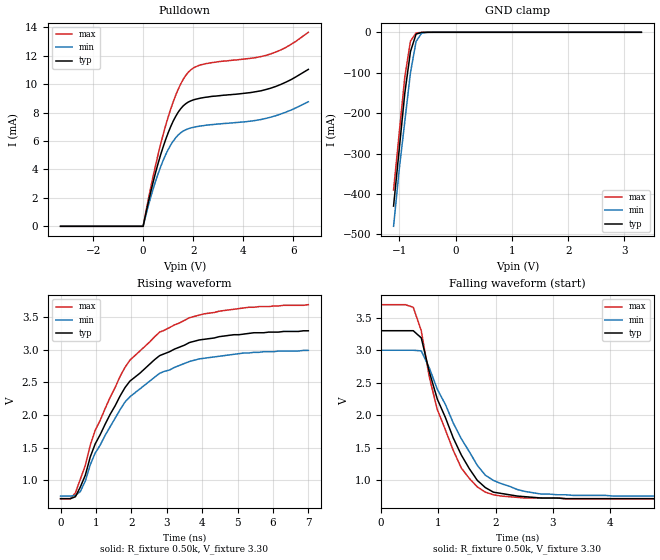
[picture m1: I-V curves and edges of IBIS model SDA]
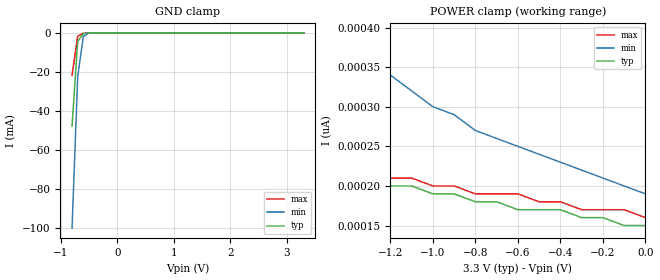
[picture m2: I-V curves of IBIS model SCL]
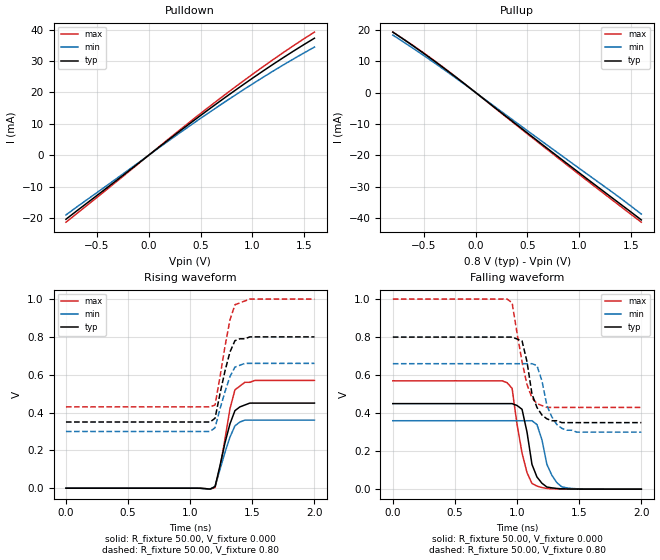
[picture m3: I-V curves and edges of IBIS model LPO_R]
| Integrated Devices Technolgy, Inc
[Ibis Ver]   3.2
[File Name]   9eprs488.ibs
[File Rev]   1.0
[Date]   08/18/2010
[Source]   Integrated Devices Technolgy, Inc.
[Notes]   Rev 0.0 created by ss
[Disclaimer] Integrated Device Technology, Inc. ("IDT") hereby grants the
   user of this IBIS model a non-exclusive, nontransferable
   license to use this IBIS model under the following terms. The
   user is granted this license only to use the IBIS model and is
   not granted rights to sell, copy (except as needed to run the
   IBIS model), rent, lease or sub-license the IBIS model in
   whole or in part, or in modified form to anyone. The User may
   modify the IBIS model to suit its specific applications, but
   rights to derivative works and such modifications shall belong
   to IDT. This IBIS model is provided on an AS IS" basis and IDT
   makes absolutely no warranty with respect to the information
   contained herein. IDT DISCLAIMS AND CUSTOMER WAIVES ALL
   WARRANTIES, EXPRESS AND IMPLIED, INCLUDING WARRANTIES OF
   MERCHANTABILITY AND FITNESS FOR A PARTICULAR PURPOSE. THE
   ENTIRE RISK AS TO QUALITY AND PERFORMANCE IS WITH THE USER
   ACCORDINGLY, IN NO EVENT SHALL IDT BE LIABLE FOR ANY DIRECT OR
   INDIRECT DAMAGES, WHETHER IN CONTRACT OR TORT, INCLUDING ANY
   LOST PROFITS OR OTHER INCIDENTAL, CONSEQUENTIAL, EXEMPLARY, OR
   PUNITIVE DAMAGES ARISING OUT OF THE USE OR APPLICATION OF THE
   IBIS model. Further, IDT reserves the right to make changes
   without notice to any product herein to improve reliability,
   function, or design. IDT does not convey any license under
   patent rights or any other intellectual property rights,
   including those of third parties. IDT is not obligated to
   provide maintenance or support for the licensed IBIS model.
[Copyright]   Copyright 2006, Integrated Devices Technolgy, Inc. all rights
   reserved
|   COMPONENT: ICS9LPRS4888
[Component]   IDT9LPRS488
[Manufacturer]   Integrated Device Technology, Inc.
[Package]
| variable   typ   min   max
R_pkg   81.1m   62.2m   100.0m
L_pkg   6.7nH   4.9nH   8.5nH
C_pkg   0.53pF   0.21pF   0.85pF
[Pin]  signal_name   model_name   R_pin   L_pin   C_pin
1   SMBCLK   SCL
2   SMBDAT   SDA
3   VDD   POWER
4   SRC7C_LPRS/27MHz_NS   LPO_R
5   SRC7T_LPRS/27MHz_SS   LPO_R
6   GND   GND
7   SRC5C_LPRS   LPO_R
8   SRC5T_LPRS   LPO_R
9   SRC4C_LPRS   LPO_R
10   SRC4T_LPRS   LPO_R
11   GNDSRC   GND
12   VDDSRC_IO   POWER
13   SRC3C_LPRS   LPO_R
14   SRC3T_LPRS   LPO_R
15   SRC2C_LPRS   LPO_R
16   SRC2T_LPRS   LPO_R
17   VDDSRC   POWER
18   VDDSRC_IO   POWER
19   GNDSRC   GND
20   SRC1C_LPRS   LPO_R
21   SRC1T_LPRS   LPO_R
22   SRC0C_LPRS   LPO_R
23   SRC0T_LPRS   LPO_R
24   **CLKREQ0#   IN_PD
25   ATIG2C_LPRS   LPO_R
26   ATIG2T_LPRS   LPO_R
27   GNDATIG   GND
28   VDDATIG_IO   POWER
29   VDDATIG   POWER
30   ATIG1C_LPRS   LPO_R
31   ATIG1T_LPRS   LPO_R
32   ATIG0C_LPRS   LPO_R
33   ATIG0T_LPRS   LPO_R
34   SB_SRC1C_LPRS   LPO_R
35   SB_SRC1T_LPRS   LPO_R
36   GNDSB_SRC   GND
37   VDDSB_SRC_IO   POWER
38   VDDSB_SRC   POWER
39   SB_SRC0C_LPRS   LPO_R
40   SB_SRC0T_LPRS   LPO_R
41   SB_SRC_SLOW#*   IN_PU
42   CLKREQ4#**   IN_PD
43   CLKREQ3#**   IN_PD
44   VDDSATA   POWER
45   SRC6C/SATAC_LPRS   LPO_R
46   SRC6T/SATAT_LPRS   LPO_R
47   GNDSATA   GND
48   GNDA   GND
49   VDDA   POWER
50   CLKREQ2#**   IN_PD
51   CLKREQ1#**   IN_PD
52   GNDCPU   GND
53   VDDCPU_IO   POWER
54   VDDCPU   POWER
55   CPUKG0C_LPR   LPO_R
56   CPUKG0T_LPRS   LPO_R
57   PD#   IN
58   GNDHTT   GND
59   HTT0C_LPRS/66M   LPO_R
60   HTT0T_LPRS/66M   LPO_R
61   VDDHTT   POWER
62   VDDREF   POWER
63   REF2/SEL_27   SE_2X_SR
64   REF1/SEL_SATA   SE_2X_SR
65   REF0/SEL_HTT66   SE_2X_SR
66   GNDREF   GND
67   X1   XT1
68   X2   XTL_OUT
69   VDD48   POWER
70   48MHz_1   SE_2X_SR
71   48MHz_0   SE_2X_SR
72   GND48   GND
[Diff Pin]   inv_pin   vdiff   tdelay_typ   tdelay_min   tdelay_max
5   4   NA   NA
8   7   NA   NA
10   9   NA   NA
14   13   NA   NA
16   15   NA   NA
21   20   NA   NA
23   22   NA   NA
26   25   NA   NA
31   30   NA   NA
33   32   NA   NA
35   34   NA   NA
40   39   NA   NA
46   45   NA   NA
56   55   NA   NA
60   59   NA   NA
| Models and submodels in the file (9): SDA (I/O_open_drain), SCL (Input), LPO_R (Output), XT1 (Input), IN (Input), SE_2X_SR (Output), IN_PD (Input), IN_PU (Input), XTL_OUT (Output)
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|   Model SDA
[Model]   SDA
Model_type   I/O_open_drain
Polarity   Inverting
Enable   Active-High
Vinl =   0.80V
Vinh =   2.00V
Vmeas =   1.50V
Cref =   5.00pF
Rref =  0.000
Vref =   1.50V
C_comp   3.40pF   2.85pF   3.95pF
[Temperature Range]   27.00   70.00   0.000
[Voltage Range]   3.30V   3.00V   3.70V
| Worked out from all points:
|   slope of the pulldown table from 0 to 0.495 V, typ, clamps not added: 131 ohm
|   GND clamp passes 1 mA (typ) near -0.62 V on its own axis
|   rising waveform, R_fixture 0.50k, V_fixture 3.30: 20-80 % time 1.74ns typ, 1.76ns min, 1.73ns max; typ from 0.72 V to 3.29 V
|   falling waveform, R_fixture 0.50k, V_fixture 3.30: 20-80 % time 693ps typ, 785ps min, 596ps max; typ from 3.3 V to 0.72 V
[Pulldown]
| voltage   I(typ)   I(min)   I(max)
-3.3V     0A         0A         0A
0V        0A         0A         0A
500mV     3.8mA      3.19mA     4.32mA
900mV     6.11mA     5.04mA     7.1mA
1.2V      7.4mA      5.99mA     8.75mA
1.4V      8.03mA     6.42mA     9.64mA
1.8V      8.74mA     6.86mA     10.83mA
2.1V      8.94mA     7mA        11.22mA
2.5V      9.08mA     7.11mA     11.44mA
5.1V      9.72mA     7.68mA     12.13mA
5.7V      10.14mA    8.03mA     12.58mA
6.6V      11.04mA    8.76mA     13.65mA
[GND_clamp]
| voltage   I(typ)   I(min)   I(max)
  |-3.30   -3.78A   -3.64A   -3.87A
  |-3.20   -3.62A   -3.50A   -3.71A
  |-3.10   -3.47A   -3.35A   -3.55A
  |-3.00   -3.31A   -3.21A   -3.39A
  |-2.90   -3.16A   -3.06A   -3.23A
  |-2.80   -3.01A   -2.91A   -3.07A
  |-2.70   -2.85A   -2.77A   -2.91A
  |-2.60   -2.70A   -2.62A   -2.75A
  |-2.50   -2.54A   -2.48A   -2.59A
  |-2.40   -2.39A   -2.33A   -2.43A
  |-2.30   -2.24A   -2.19A   -2.27A
  |-2.20   -2.08A   -2.04A   -2.11A
  |-2.10   -1.93A   -1.90A   -1.95A
  |-2.00   -1.78A   -1.75A   -1.79A
  |-1.90   -1.62A   -1.61A   -1.63A
  |-1.80   -1.47A   -1.46A   -1.47A
  |-1.70   -1.32A   -1.32A   -1.32A
  |-1.60   -1.17A   -1.18A   -1.16A
  |-1.50   -1.02A   -1.03A   -1.00A
  |-1.40   -0.87A   -0.89A   -0.85A
  |-1.30   -0.72A   -0.75A   -0.69A
  |-1.20   -0.57A   -0.61A   -0.54A
-1.1V     -430mA     -480mA     -390mA
-1V       -290mA     -340mA     -250mA
-900mV    -150mA     -220mA     -110mA
-800mV    -47.73mA   -100mA     -21.74mA
-700mV    -4.4mA     -22.46mA   -1.7mA
-600mV    -390uA     -1.82mA    -190uA
-400mV    -1.59uA    -9.25uA    -420nA
3.3V      150pA      220pA      150pA
[Ramp]
| variable   typ   min   max
dV/dt_r   0.27/0.19n   0.21/0.19n   0.35/0.18n
dV/dt_f   0.27/0.21n   0.21/0.22n   0.35/0.20n
[Rising Waveform]
R_fixture = 0.50k
V_fixture = 3.30
V_fixture_min = 3.00
V_fixture_max = 3.70
| time   V(typ)   V(min)   V(max)
0s        720mV      760mV      720mV
280ps     720mV      760mV      720mV
420ps     750mV      770mV      810mV
560ps     900mV      830mV      1.02V
700ps     1.08V      990mV      1.23V
980ps     1.56V      1.42V      1.77V
1.82ns    2.42V      2.2V       2.73V
2.8ns     2.91V      2.64V      3.27V
4.06ns    3.16V      2.87V      3.55V
7ns       3.29V      2.99V      3.69V
[Falling Waveform]
R_fixture = 0.50k
V_fixture = 3.30
V_fixture_min = 3.00
V_fixture_max = 3.70
| time   V(typ)   V(min)   V(max)
0s        3.3V       3V         3.7V
560ps     3.3V       3V         3.66V
700ps     3.19V      2.99V      3.3V
840ps     2.67V      2.73V      2.59V
980ps     2.25V      2.4V       2.09V
1.4ns     1.39V      1.64V      1.19V
1.68ns    1V         1.23V      900mV
1.82ns    890mV      1.08V      820mV
2.8ns     730mV      790mV      730mV
7ns       720mV      760mV      720mV
|   Model SCL
[Model]   SCL
Model_type   Input
Polarity   Non-Inverting
Enable   Active-High
Vinl =   0.80V
Vinh =   2.00V
C_comp   3.40pF   2.85pF   3.95pF
[Temperature Range]   27.00   70.00   0.000
[Voltage Range]   3.30V   3.00V   3.60V
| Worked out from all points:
|   GND clamp passes 1 mA (typ) near -0.62 V on its own axis
[GND_clamp]
| voltage   I(typ)   I(min)   I(max)
|  -3.30   -3.78A   -3.64A   -3.87A
|  -3.20   -3.62A   -3.50A   -3.71A
|  -3.10   -3.47A   -3.35A   -3.55A
|  -3.00   -3.31A   -3.21A   -3.39A
|  -2.90   -3.16A   -3.06A   -3.23A
|  -2.80   -3.01A   -2.91A   -3.07A
|  -2.70   -2.85A   -2.77A   -2.91A
|  -2.60   -2.70A   -2.62A   -2.75A
|  -2.50   -2.54A   -2.48A   -2.59A
|  -2.40   -2.39A   -2.33A   -2.43A
|  -2.30   -2.24A   -2.19A   -2.27A
|  -2.20   -2.08A   -2.04A   -2.11A
|  -2.10   -1.93A   -1.90A   -1.95A
|  -2.00   -1.78A   -1.75A   -1.79A
|  -1.90   -1.62A   -1.61A   -1.63A
|  -1.80   -1.47A   -1.46A   -1.47A
|  -1.70   -1.32A   -1.32A   -1.32A
|  -1.60   -1.17A   -1.18A   -1.16A
|  -1.50   -1.02A   -1.03A   -1.00A
|  -1.40   -0.87A   -0.89A   -0.85A
|  -1.30   -0.72A   -0.75A   -0.69A
|  -1.20   -0.57A   -0.61A   -0.54A
|  -1.10   -0.43A   -0.48A   -0.39A
|  -1.00   -0.29A   -0.34A   -0.25A
|  -0.90   -0.15A   -0.22A   -0.11A
-800mV    -47.73mA   -100mA     -21.74mA
-700mV    -4.4mA     -22.46mA   -1.7mA
-600mV    -390uA     -1.82mA    -190uA
-500mV    -33.11uA   -140uA     -13.41uA
-400mV    -1.59uA    -9.25uA    -420nA
3.3V      150pA      220pA      150pA
[POWER_clamp]
| voltage   I(typ)   I(min)   I(max)
-3.3V     350pA      1.67nA     300pA
-2.6V     280pA      890pA      270pA
-2.5V     280pA      820pA      260pA
-2.3V     260pA      700pA      260pA
-2.2V     250pA      640pA      250pA
-1.5V     220pA      400pA      220pA
-1.4V     210pA      380pA      220pA
-1V       190pA      300pA      200pA
-800mV    180pA      270pA      190pA
-600mV    170pA      250pA      190pA
-400mV    170pA      230pA      180pA
0V        150pA      190pA      160pA
|   Model LPO_R
[Model]   LPO_R
Model_type   Output
Polarity   Inverting
Vmeas =   0.40V
Cref =   2.00pF
Rref =  0.000
Vref =   0.40V
C_comp   3.40pF   2.85pF   3.95pF
[Temperature Range]   27.00   70.00   0.000
[Voltage Range]   0.80V   0.66V   1.00V
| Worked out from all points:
|   slope of the pulldown table from 0 to 0.12 V, typ, clamps not added: 38.7 ohm
|   slope of the pullup table from 0 to 0.12 V, typ, clamps not added: 38.5 ohm
|   rising waveform, R_fixture 50.00, V_fixture 0.000: 20-80 % time 102ps typ, 104ps min, 93.3ps max; typ from 0 V to 0.45 V
|   rising waveform, R_fixture 50.00, V_fixture 0.80: 20-80 % time 94.5ps typ, 98.2ps min, 91.1ps max; typ from 0.35 V to 0.8 V
|   falling waveform, R_fixture 50.00, V_fixture 0.000: 20-80 % time 84.2ps typ, 95.2ps min, 93.9ps max; typ from 0.45 V to 0 V
|   falling waveform, R_fixture 50.00, V_fixture 0.80: 20-80 % time 88.8ps typ, 97ps min, 99.9ps max; typ from 0.8 V to 0.35 V
[Pulldown]
| voltage   I(typ)   I(min)   I(max)
-800mV    -20.43mA   -19.07mA   -21.37mA
200mV     5.15mA     4.77mA     5.4mA
700mV     17.5mA     16.21mA    18.38mA
1.2V      28.96mA    26.79mA    30.45mA
1.6V      37.29mA    34.46mA    39.24mA
[Pullup]
| voltage   I(typ)   I(min)   I(max)
-800mV    19.3mA     18.34mA    19.28mA
-600mV    14.81mA    14.03mA    14.91mA
-300mV    7.63mA     7.2mA      7.75mA
800mV     -20.57mA   -19.4mA    -20.99mA
1.4V      -35.64mA   -33.74mA   -36.34mA
1.6V      -40.66mA   -38.79mA   -41.38mA
[Ramp]
| variable   typ   min   max
dV/dt_r   0.27/83.86p   0.22/88.13p   0.34/83.56p
dV/dt_f   0.27/85.35p   0.21/93.50p   0.34/84.82p
[Rising Waveform]
R_fixture = 50.00
V_fixture = 0.000
V_fixture_min = 0.000
V_fixture_max = 0.000
| time   V(typ)   V(min)   V(max)
0s        0V         0V         0V
1.16ns    -4.69mV    -5.01mV    -4.52mV
1.2ns     7.99mV     10.25mV    3.07mV
1.24ns    120mV      99.58mV    110mV
1.28ns    240mV      190mV      260mV
1.32ns    340mV      270mV      420mV
1.36ns    410mV      330mV      520mV
1.44ns    440mV      360mV      560mV
1.52ns    450mV      360mV      570mV
2ns       450mV      360mV      570mV
[Rising Waveform]
R_fixture = 50.00
V_fixture = 0.80
V_fixture_min = 0.66
V_fixture_max = 1.00
| time   V(typ)   V(min)   V(max)
0s        350mV      300mV      430mV
1.16ns    350mV      300mV      430mV
1.2ns     370mV      320mV      440mV
1.24ns    500mV      420mV      590mV
1.28ns    620mV      510mV      750mV
1.32ns    720mV      590mV      890mV
1.36ns    780mV      640mV      970mV
1.44ns    790mV      660mV      990mV
1.48ns    800mV      660mV      1V
2ns       800mV      660mV      1V
[Falling Waveform]
R_fixture = 50.00
V_fixture = 0.000
V_fixture_min = 0.000
V_fixture_max = 0.000
| time   V(typ)   V(min)   V(max)
0s        450mV      360mV      570mV
920ps     450mV      360mV      560mV
960ps     450mV      360mV      530mV
1.04ns    420mV      360mV      190mV
1.12ns    130mV      360mV      30.02mV
1.16ns    64mV       340mV      16.44mV
1.2ns     31.2mV     260mV      8.36mV
1.24ns    11.25mV    130mV      3.88mV
1.36ns    1.85mV     12.17mV    770uV
2ns       23.17uV    48.72uV    15.23uV
[Falling Waveform]
R_fixture = 50.00
V_fixture = 0.80
V_fixture_min = 0.66
V_fixture_max = 1.00
| time   V(typ)   V(min)   V(max)
0s        800mV      660mV      1V
920ps     800mV      660mV      1V
960ps     800mV      660mV      980mV
1.04ns    780mV      660mV      670mV
1.08ns    670mV      660mV      550mV
1.12ns    500mV      660mV      480mV
1.16ns    430mV      650mV      450mV
1.24ns    370mV      440mV      430mV
1.36ns    350mV      320mV      430mV
2ns       350mV      300mV      430mV
